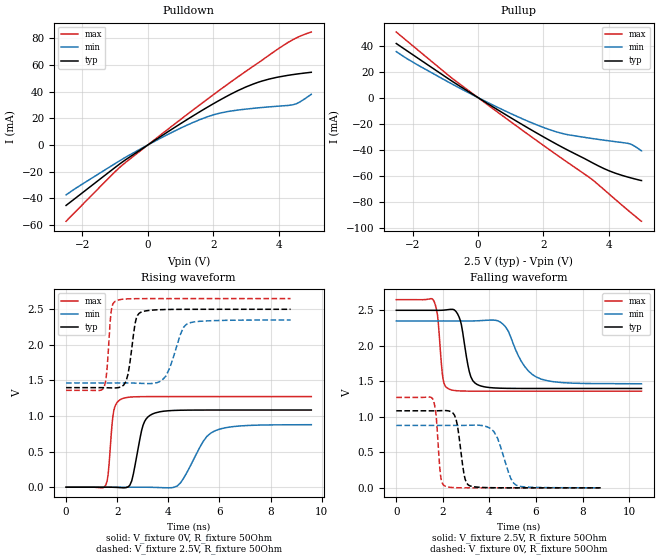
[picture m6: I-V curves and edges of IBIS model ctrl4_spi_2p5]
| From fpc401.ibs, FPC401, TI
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|   ctrl4_spi_2p5 Model
[Model]   ctrl4_spi_2p5
Model_type   Output
Polarity   Non-Inverting
Vmeas = 1.25
Vref = 0
Cref = 2pF
Rref = 100
|   typ   min   max
|   (nom PVT)   (fast PVT)   (slow PVT)
C_comp   1.233e-14   1.168e-14   1.967e-14
| Where nom  PVT is Nominal Process, 2.5V, 27C
|   Fast PVT is Strong Process,  2.65V, -40C
|   Slow PVT is Weak Process,   2.35V, 125C
[Voltage Range]   2.5   2.35   2.65
|Junction Temperature
[Temperature Range]   27   125   -40
[Pullup Reference]   2.5   2.35   2.65
[Pulldown Reference]   0   0   0
[Power Clamp Reference]   2.5   2.35   2.65
[GND Clamp Reference]   0   0   0
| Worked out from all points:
|   slope of the pulldown table from 0 to 0.375 V, typ, clamps not added: 61.9 ohm
|   slope of the pullup table from 0 to 0.375 V, typ, clamps not added: 63.9 ohm
|   falling waveform, V_fixture 2.5V, R_fixture 50Ohm: 20-80 % time 346ps typ, 836ps min, 191ps max; typ from 2.5 V to 1.4 V
|   rising waveform, V_fixture 0V, R_fixture 50Ohm: 20-80 % time 360ps typ, 808ps min, 176ps max; typ from 0 V to 1.08 V
|   rising waveform, V_fixture 2.5V, R_fixture 50Ohm: 20-80 % time 251ps typ, 493ps min, 152ps max; typ from 1.4 V to 2.5 V
|   falling waveform, V_fixture 0V, R_fixture 50Ohm: 20-80 % time 265ps typ, 524ps min, 166ps max; typ from 1.08 V to 0 V
[Pulldown]
|   Voltage   I(typ)   I(min)   I(max)
-2.5V     -45.19mA   -37.31mA   -57.06mA
-748.3mV  -12.19mA   -10.12mA   -14.37mA
350mV     5.699mA    4.606mA    6.76mA
1.208V    19.16mA    14.97mA    22.98mA
1.782V    27.72mA    20.77mA    33.6mA
2.271V    34.55mA    24.21mA    42.43mA
2.755V    40.71mA    26.17mA    50.98mA
3.377V    46.97mA    27.82mA    61.51mA
3.932V    50.58mA    28.97mA    71.07mA
4.437V    52.7mA     30.1mA     78.83mA
4.646V    53.4mA     32.19mA    81.34mA
5V        54.44mA    37.94mA    84.54mA
[Pullup]
|   Voltage   I(typ)   I(min)   I(max)
-2.5V     41.57mA    35.32mA    50.39mA
-1.833V   30.17mA    24.87mA    36.41mA
-584.7mV  9.218mA    7.568mA    10.92mA
747.7mV   -11.66mA   -9.309mA   -13.97mA
1.74V     -26.5mA    -20.43mA   -32.12mA
2.24V     -33.62mA   -25.12mA   -41.09mA
2.635V    -39mA      -27.99mA   -48.07mA
3.505V    -50.27mA   -31.55mA   -63.33mA
3.855V    -54.68mA   -32.79mA   -70.84mA
4.6V      -61.29mA   -35.33mA   -86.98mA
4.753V    -62.32mA   -36.87mA   -90.17mA
5V        -63.87mA   -40.95mA   -95.18mA
[Ramp]
R_load = 50
|   typ   min   max
dV/dt_r   0.650802/3.60339e-10   0.527276/8.08711e-10   0.764069/1.76138e-10
dV/dt_f   0.660539/3.46457e-10   0.531059/8.35959e-10   0.773301/1.90909e-10
[Falling Waveform]
V_fixture = 2.5V
V_fixture_min = 2.35V
V_fixture_max = 2.65V
R_fixture = 50Ohm
|   Time   V(typ)   V(min)   V(max)
0s        2.5V       2.35V      2.65V
1.604ns   2.5V       2.35V      2.638V
1.773ns   2.499V     2.35V      2.424V
2.011ns   2.502V     2.35V      1.527V
2.322ns   2.513V     2.35V      1.383V
2.695ns   2.407V     2.35V      1.365V
3.561ns   1.443V     2.353V     1.361V
4.599ns   1.402V     2.301V     1.361V
6.23ns    1.399V     1.53V      1.361V
10.53ns   1.399V     1.465V     1.361V
[Rising Waveform]
V_fixture = 0V
V_fixture_min = 0V
V_fixture_max = 0V
R_fixture = 50Ohm
|   Time   V(typ)   V(min)   V(max)
0s        566.4pV    16.09nV    343.2pV
1.555ns   420.2uV    52.21nV    31.24mV
1.869ns   -958.3uV   2.973uV    1.078V
2.193ns   -7.376mV   -22.74uV   1.243V
2.569ns   90.03mV    271.5uV    1.268V
3.012ns   872.2mV    313.2uV    1.273V
3.381ns   1.029V     -1.59mV    1.273V
4.35ns    1.08V      17.79mV    1.274V
5.844ns   1.085V     795.8mV    1.274V
9.594ns   1.085V     878.5mV    1.274V
[Rising Waveform]
V_fixture = 2.5V
V_fixture_min = 2.35V
V_fixture_max = 2.65V
R_fixture = 50Ohm
|   Time   V(typ)   V(min)   V(max)
0s        1.399V     1.465V     1.361V
1.499ns   1.399V     1.465V     1.416V
1.773ns   1.396V     1.465V     2.492V
2.011ns   1.398V     1.465V     2.627V
2.343ns   1.485V     1.465V     2.645V
2.695ns   2.294V     1.463V     2.649V
2.955ns   2.463V     1.459V     2.65V
3.906ns   2.497V     1.563V     2.65V
4.821ns   2.5V       2.308V     2.65V
8.783ns   2.5V       2.35V      2.65V
[Falling Waveform]
V_fixture = 0V
V_fixture_min = 0V
V_fixture_max = 0V
R_fixture = 50Ohm
|   Time   V(typ)   V(min)   V(max)
0s        1.085V     878.8mV    1.274V
1.555ns   1.084V     878.8mV    1.258V
1.715ns   1.085V     878.8mV    1.006V
1.9ns     1.086V     878.8mV    178mV
2.104ns   1.088V     878.8mV    23.32mV
2.569ns   965.3mV    878.6mV    2.022mV
3.136ns   31.46mV    881mV      161.6uV
4.188ns   1.639mV    794.7mV    -2.411uV
5.13ns    196.4uV    41.55mV    9.453uV
8.783ns   -1.241uV   264.9uV    16.89uV
